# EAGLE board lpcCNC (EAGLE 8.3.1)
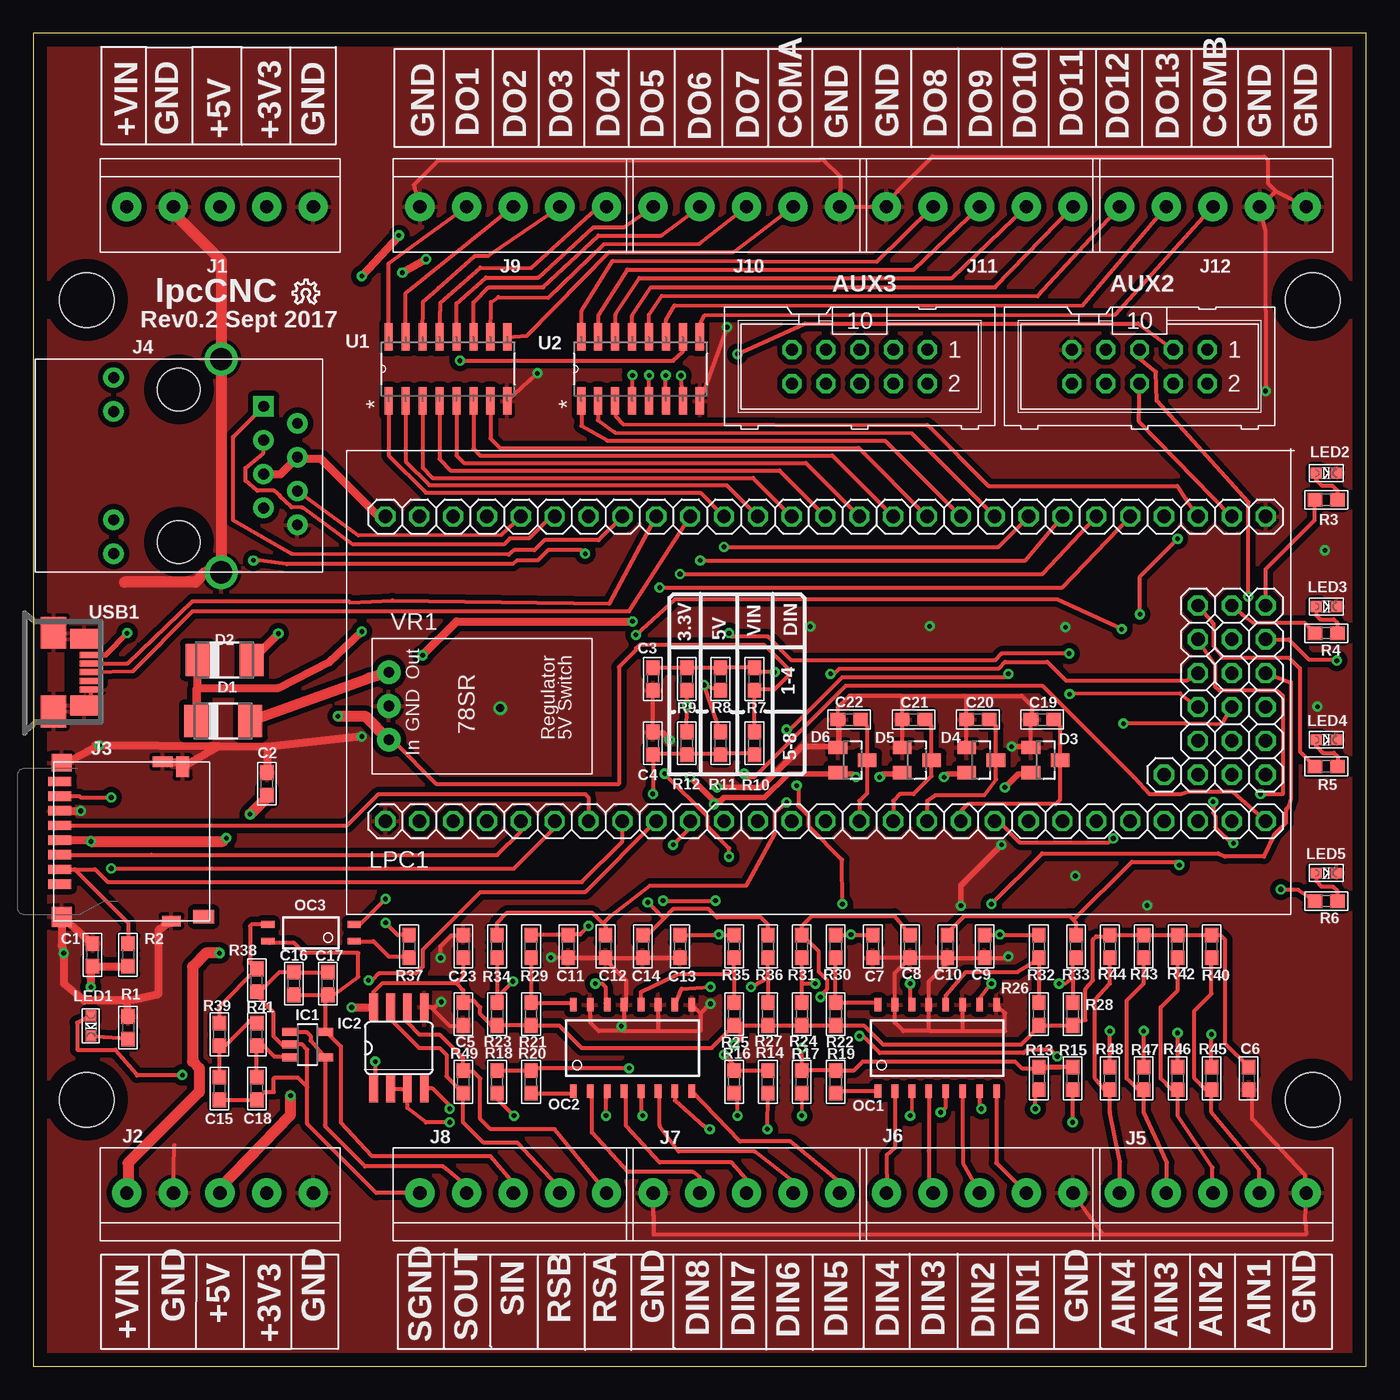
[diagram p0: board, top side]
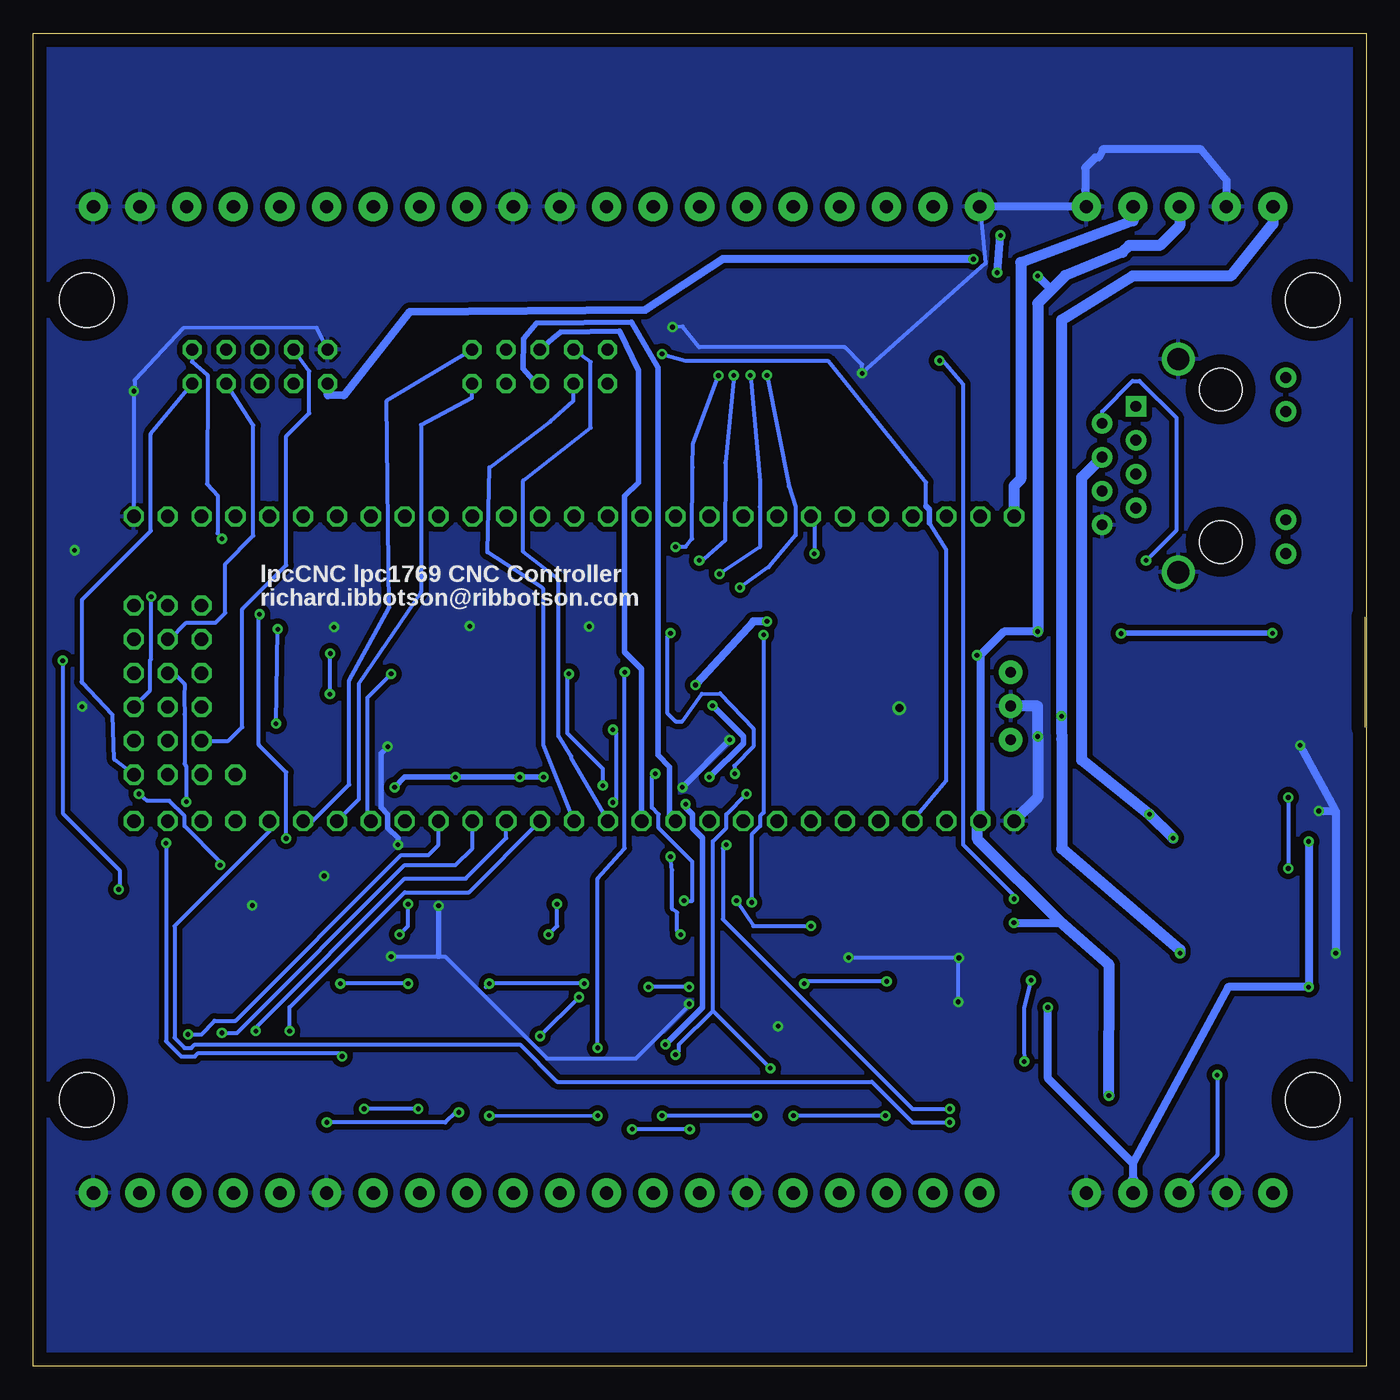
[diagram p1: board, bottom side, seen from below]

Size 100 x 100 mm. Coordinates in mm from the lower left corner, seen from the top.
Outline: 0,0 100,0 100,100 0,100 0,0
Copper layers (1*16): Top 0.035mm / dielectric 1.5mm / Bottom 0.035mm
Design rules "pcbway": minimum track width 6mil, minimum drill 0.3mm, track to track 0.205mm, track to pad 0.205mm, pad to pad 0.205mm, via to via 0.205mm, smd to smd 8mil, copper to edge 40mil, drill to drill 8mil, minimum pad ring 10mil, minimum via ring 8mil, stop-mask expansion 4mil, vias tented up to drill 25mil, thermal gap 10mil
Holes 4.1 mm at 4,20 96,20 96,80 4,80

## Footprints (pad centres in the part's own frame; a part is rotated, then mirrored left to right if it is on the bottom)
ML10 = drill 0.914 octagon: 1 -5.08,-1.27; 2 -5.08,1.27; 3 -2.54,-1.27; 4 -2.54,1.27; 5 0,-1.27; 6 0,1.27; 7 2.54,-1.27; 8 2.54,1.27; 9 5.08,-1.27; 10 5.08,1.27
0603 = smd 1.1 x 1: 1 -0.85,0; 2 0.85,0
DO-214AC = smd 1.8 x 2.4: A 2.025,0; C -2.025,0
SOT23 = smd 1 x 1.4: 1 -0.95,-1.1; 2 0.95,-1.1; 3 0,1.1
SOT23-5 = smd 0.6 x 1.2: 1 -0.95,-1.306; 2 0,-1.306; 3 0.95,-1.306; 4 0.95,1.306; 5 -0.95,1.306
SO08 = smd 0.66 x 2.032: 1 -1.905,-3.073; 2 -0.635,-3.073; 3 0.635,-3.073; 4 1.905,-3.073; 5 1.905,3.073; 6 0.635,3.073; 7 -0.635,3.073; 8 -1.905,3.073
1X05-3.5MM = drill 1 pad 2.184: 1 7,0; 2 3.5,0; 3 0,0; 4 -3.5,0; 5 -7,0
AMPHENOL_114-00841-68 = smd 0.7 x 1.75: 1 3.2,-5.888; 2 2.1,-5.888; 3 1,-5.888; 4 -0.1,-5.888; 5 -1.2,-5.888; 6 -2.3,-5.888; 7 -3.4,-5.888; 8 -4.5,-5.888 | smd 1 x 1.55: CD1 5.65,4.912 | smd 1.55 x 1: CD2 -5.602,3.337 | smd 1.3 x 1.5: SH1 -5.9,-5.76 | smd 1.5 x 1.5: SH2 5.65,-5.76 | smd 0.8 x 1.4: SH3 5.975,2.487 | smd 0.8 x 1.5: SH4 -5.975,1.837
HR911105A = drill 0.813 pad 1.524 square: 1 4.445,-6.35 | drill 0.813 pad 1.524: 2 3.175,-8.89; 3 1.905,-6.35; 4 0.635,-8.89; 5 -0.635,-6.35; 6 -1.905,-8.89; 7 -3.175,-6.35; 8 -4.445,-8.89; 9 6.604,4.902; 10 4.064,4.902; 11 -4.064,4.902; 12 -6.604,4.902 | drill 1.651 pad 2.159: 13 8.001,-3.175; 14 -8.001,-3.175 | hole 3.2: 5.715,0; -5.715,0
CHIPLED_0603 = smd 0.8 x 0.8: A 0,-0.75; C 0,0.75
LPCXPRESSO_LPC1769 = drill 1 octagon: 1 -0.635,-10.795; 2 1.905,-10.795; 3 4.445,-10.795; 4 6.985,-10.795; 5 9.525,-10.795; 6 12.065,-10.795; 7 14.605,-10.795; 8 17.145,-10.795; 9 19.685,-10.795; 10 22.225,-10.795; 11 24.765,-10.795; 12 27.305,-10.795; 13 29.845,-10.795; 14 32.385,-10.795; 15 34.925,-10.795; 16 37.465,-10.795; 17 40.005,-10.795; 18 42.545,-10.795; 19 45.085,-10.795; 20 47.625,-10.795; 21 50.165,-10.795; 22 52.705,-10.795; 23 55.245,-10.795; 24 57.785,-10.795; 25 60.325,-10.795; 26 62.865,-10.795; 27 65.405,-10.795; 28 -0.635,12.065; 29 1.905,12.065; 30 4.445,12.065; 31 6.985,12.065; 32 9.525,12.065; 33 12.065,12.065; 34 14.605,12.065; 35 17.145,12.065; 36 19.685,12.065; 37 22.225,12.065; 38 24.765,12.065; 39 27.305,12.065; 40 29.845,12.065; 41 32.385,12.065; 42 34.925,12.065; 43 37.465,12.065; 44 40.005,12.065; 45 42.545,12.065; 46 45.085,12.065; 47 47.625,12.065; 48 50.165,12.065; 49 52.705,12.065; 50 55.245,12.065; 51 57.785,12.065; 52 60.325,12.065; 53 62.865,12.065; 54 65.405,12.065; 55 57.785,-7.315; 56 60.325,-7.315; 57 62.865,-7.315; 58 65.405,-7.315; 59 60.325,-4.775; 60 62.865,-4.775; 61 65.405,-4.775; 62 60.325,-2.235; 63 62.865,-2.235; 64 65.405,-2.235; 65 60.325,0.305; 66 62.865,0.305; 67 65.405,0.305; 68 60.325,2.845; 69 62.865,2.845; 70 65.405,2.845; 71 60.325,5.385; 72 62.865,5.385; 73 65.405,5.385
MINI-FLAT-16 = smd 1 x 0.5: 1 -3.24,4.445; 2 -3.24,3.175; 3 -3.24,1.905; 4 -3.24,0.635; 5 -3.24,-0.635; 6 -3.24,-1.905; 7 -3.24,-3.175; 8 -3.24,-4.445; 9 3.24,-4.445; 10 3.24,-3.175; 11 3.24,-1.905; 12 3.24,-0.635; 13 3.24,0.635; 14 3.24,1.905; 15 3.24,3.175; 16 3.24,4.445
MINI-FLAT-4 = smd 1 x 0.5: 1 -3.24,0.635; 2 -3.24,-0.635; 3 3.24,-0.635; 4 3.24,0.635
SOIC127P600X175-16N = smd 2.057 x 0.61: 1 -4.801,8.89; 2 -4.801,7.62; 3 -4.801,6.35; 4 -4.801,5.08; 5 -4.801,3.81; 6 -4.801,2.54; 7 -4.801,1.27; 8 -4.801,0; 9 0,0; 10 0,1.27; 11 0,2.54; 12 0,3.81; 13 0,5.08; 14 0,6.35; 15 0,7.62; 16 0,8.89
MOLEX-47364-0001 = smd 1.7 x 0.45: 1 2.8,1.3; 2 2.8,0.65; 3 2.8,0; 4 2.8,-0.65; 5 2.8,-1.3 | smd 1.9 x 2.375: GND1 0,2.95; GND4 0,-2.95 | smd 2.1 x 1.475: GND2 2.3,2.5; GND3 2.3,-2.5
78SR = drill 0.8 pad 1.778: P1 -2.54,0; P2 0,0; P3 2.54,0

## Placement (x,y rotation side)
AUX2  [ML10]  83,75 180 top
AUX3  [ML10]  62,75 180 top
C1  100n  [0603]  4.45,30.86 90 top
C2  100n  [0603]  17.53,43.69 90 top
C3  100n  [0603]  46.48,51.56 270 top
C4  100n  [0603]  46.48,46.74 90 top
C5  100n  [0603]  32.26,26.42 270 top
C6  100n  [0603]  91.19,21.59 270 top
C7  100n  [0603]  62.99,31.5 270 top
C8  100n  [0603]  65.79,31.5 270 top
C9  100n  [0603]  71.37,31.5 270 top
C10  100n  [0603]  68.58,31.5 270 top
C11  100n  [0603]  40.13,31.5 270 top
C12  100n  [0603]  42.93,31.5 270 top
C13  100n  [0603]  48.51,31.5 270 top
C14  100n  [0603]  45.72,31.5 270 top
C15  47n  [0603]  13.97,20.83 270 top
C16  1uF  [0603]  19.56,28.7 90 top
C17  100n  [0603]  22.1,28.7 90 top
C18  100n  [0603]  16.76,20.83 270 top
C19  1uF  [0603]  75.69,48.51 180 top
C20  1uF  [0603]  70.87,48.51 180 top
C21  1uF  [0603]  66.04,48.51 180 top
C22  1uF  [0603]  61.21,48.51 180 top
C23  100n  [0603]  32.26,31.5 90 top
D1  [DO-214AC]  14.35,52.98 0 top
D2  [DO-214AC]  14.25,48.41 0 top
D3  BAS70  [SOT23]  75.95,45.47 270 top
D4  BAS70  [SOT23]  71.12,45.47 270 top
D5  BAS70  [SOT23]  66.29,45.47 270 top
D6  BAS70  [SOT23]  61.47,45.47 270 top
IC1  TLV172  [SOT23-5]  20.57,24.13 270 top
IC2  MAX3485  [SO08]  27.43,23.88 0 top
J1  1X5  [1X05-3.5MM]  14,87 180 top
J2  1X5  [1X05-3.5MM]  14,13 0 top
J3  [AMPHENOL_114-00841-68]  7.87,39.37 270 top
J4  HR911105A  [HR911105A]  10.92,67.56 90 top
J5  1X5  [1X05-3.5MM]  88.5,13 0 top
J6  1X5  [1X05-3.5MM]  71,13 0 top
J7  1X5  [1X05-3.5MM]  53.5,13 0 top
J8  1X5  [1X05-3.5MM]  36,13 0 top
J9  1X5  [1X05-3.5MM]  36,87 180 top
J10  1X5  [1X05-3.5MM]  53.5,87 180 top
J11  1X5  [1X05-3.5MM]  71,87 180 top
J12  1X5  [1X05-3.5MM]  88.5,87 180 top
LED1  [CHIPLED_0603]  4.32,25.53 180 top
LED2  [CHIPLED_0603]  97,67 270 top
LED3  [CHIPLED_0603]  97,57 270 top
LED4  [CHIPLED_0603]  97,47 270 top
LED5  [CHIPLED_0603]  97,37 270 top
LPC1  [LPCXPRESSO_LPC1769]  27.05,51.69 0 top
OC1  TLP293-4  [MINI-FLAT-16]  67.82,23.88 90 top
OC2  TLP293-4  [MINI-FLAT-16]  44.96,23.88 90 top
OC3  OCPL217-500E  [MINI-FLAT-4]  20.83,32.51 180 top
R1  1K  [0603]  7.11,25.4 270 top
R2  100K  [0603]  7.11,30.86 270 top
R3  1K  [0603]  97,65 0 top
R4  1K  [0603]  97,55 0 top
R5  1K  [0603]  97,45 0 top
R6  1K  [0603]  97,34.9 0 top
R7  DNF  [0603]  54.1,51.56 270 top
R8  0R  [0603]  51.56,51.56 270 top
R9  DNF  [0603]  49.02,51.56 270 top
R10  DNF  [0603]  54.1,46.74 90 top
R11  0R  [0603]  51.56,46.74 90 top
R12  DNF  [0603]  49.02,46.74 90 top
R13  470R  [0603]  75.44,21.59 90 top
R14  470R  [0603]  55.12,21.34 90 top
R15  470R  [0603]  77.98,21.59 90 top
R16  470R  [0603]  52.58,21.34 90 top
R17  470R  [0603]  57.66,21.34 90 top
R18  470R  [0603]  34.8,21.34 90 top
R19  470R  [0603]  60.2,21.34 90 top
R20  470R  [0603]  37.34,21.34 90 top
R21  2K2  [0603]  37.34,26.42 270 top
R22  2K2  [0603]  60.2,26.42 270 top
R23  2K2  [0603]  34.8,26.42 270 top
R24  2K2  [0603]  57.66,26.42 270 top
R25  2K2  [0603]  52.58,26.42 270 top
R26  2K2  [0603]  75.44,26.42 270 top
R27  2K2  [0603]  55.12,26.42 270 top
R28  2K2  [0603]  77.98,26.42 270 top
R29  1K  [0603]  37.34,31.5 90 top
R30  1K  [0603]  60.2,31.5 270 top
R31  1K  [0603]  57.66,31.5 270 top
R32  1K  [0603]  75.44,31.5 270 top
R33  1K  [0603]  78.23,31.5 270 top
R34  1K  [0603]  34.8,31.5 90 top
R35  1K  [0603]  52.58,31.5 90 top
R36  1K  [0603]  55.12,31.5 90 top
R37  470R  [0603]  28.19,31.5 270 top
R38  2K2  [0603]  16.76,28.96 90 top
R39  47K  [0603]  13.97,24.89 90 top
R40  4K7  [0603]  88.39,31.5 90 top
R41  100K  [0603]  16.76,24.89 90 top
R42  4K7  [0603]  85.85,31.5 90 top
R43  4K7  [0603]  83.31,31.5 90 top
R44  4K7  [0603]  80.77,31.5 90 top
R45  10K  [0603]  88.39,21.59 270 top
R46  10K  [0603]  85.85,21.59 270 top
R47  10K  [0603]  83.31,21.59 270 top
R48  10K  [0603]  80.77,21.59 270 top
R49  120R  [0603]  32.26,21.34 270 top
U1  ULQ2003  [SOIC127P600X175-16N]  35.56,77.22 90 top
U2  ULQ2003  [SOIC127P600X175-16N]  50,77.22 90 top
U$1  [OSHW_8X70_NOTEXT]  19.46,79.73 0 top
USB1  MOLEX-47346-0001  [MOLEX-47364-0001]  1.52,52.07 0 top
VR1  78SR  [78SR]  26.67,49.53 270 top

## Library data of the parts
AUX2 AUX3 = con-ml; OC_FARNELL: unknown; OC_NEWARK: unknown
C1-C23 LED1-LED5 R1-R49 = microbuilder
D1-D6 = diode
IC1 J3 J4 LPC1 VR1 = CNClib
IC2 = maxim; MF: MAXIM; MPN: MAX481CSA; OC_FARNELL: unknown; OC_NEWARK: 90C3817
J1 J2 J5-J12 = adafruit
OC1-OC3 = optocoupler; OC_FARNELL: unknown; OC_NEWARK: unknown
U1 U2 = Texas Instruments_By_element14_Batch_1; MPN: ULN2003ADE4; OC_FARNELL: 1125398; OC_NEWARK: 93K1078; PACKAGE: SOIC-16; SUPPLIER: Texas Instruments
U$1 = ohw-logo
USB1 = usb_con-update

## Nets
+3V3: C1.1 C2.1 C5.1 C6.1 C23.1 D3.2 D4.2 D5.2 D6.2 IC2.8 J1.4 J2.2 J3.4 J4.4 J4.5 LPC1.28 R2.2 R9.2 R12.2 R21.2 R22.2 R23.2 R24.2 R25.2 R26.2 R27.2 R28.2 R40.2 R42.2 R43.2 R44.2
+5V: AUX2.10 D1.C D2.C J1.3 J2.3 LED1.A LPC1.2 R8.2 R11.2 R37.1
+12V: J1.1 J2.5 R7.2 R10.2 VR1.P3
ANI1: J5.2 R40.1 R45.2
ANI2: J5.3 R42.1 R46.2
ANI3: J5.4 R43.1 R47.2
ANI4: J5.5 R44.1 R48.2
DI1: J6.2 OC1.8
DI2: J6.3 OC1.6
DI3: J6.4 OC1.4
DI4: J6.5 OC1.2
DI5: J7.1 OC2.8
DI6: J7.2 OC2.6
DI7: J7.3 OC2.4
DI8: J7.4 OC2.2
DO1: J9.2 U1.16
DO2: J9.3 U1.15
DO3: J9.4 U1.14
DO4: J9.5 U1.13
DO5: J10.1 U1.12
DO6: J10.2 U1.11
DO7: J10.3 U1.10
DO8: J11.2 U2.16
DO9: J11.3 U2.15
DO10: J11.4 U2.14
DO11: J11.5 U2.13
DO12: J12.1 U2.12
DO13: J12.2 U2.11
ERDN: J4.6 LPC1.32
ERDP: J4.3 LPC1.33
ETDN: J4.2 LPC1.34
ETDP: J4.1 LPC1.35
GND: AUX2.9 C1.2 C2.2 C3.2 C4.2 C5.2 C6.2 C7.2 C8.2 C9.2 C10.2 C11.2 C12.2 C13.2 C14.2 C19.2 C20.2 C21.2 C22.2 C23.2 D3.1 D4.1 D5.1 D6.1 IC2.5 J1.2 J1.5 J2.1 J2.4 J3.6 J3.CD2 J3.SH1 J3.SH2 J3.SH3 J3.SH4 J4.8 J4.13 J4.14 J5.1 J6.1 J7.5 J9.1 J10.5 J11.1 J12.4 J12.5 LED2.C LED3.C LED4.C LED5.C LPC1.1 LPC1.54 OC1.9 OC1.11 OC1.13 OC1.15 OC2.9 OC2.11 OC2.13 OC2.15 R1.1 U1.8 U2.8 USB1.5 USB1.GND1 USB1.GND2 USB1.GND3 USB1.GND4 VR1.P2
N$1: D2.A VR1.P1
N$2: LED2.A R3.2
N$3: LED3.A R4.2
N$4: LED4.A R5.2
N$5: LED5.A R6.2
N$6: LED1.C R1.2
N$9: J10.4 U1.9
N$13: J12.3 U2.9
N$15: C3.1 R7.1 R8.1 R9.1 R13.2 R15.2 R17.2 R19.2
N$16: OC2.1 R20.1
N$31: OC2.3 R18.1
N$32: OC2.5 R16.1
N$33: OC2.7 R14.1
N$38: C4.1 R10.1 R11.1 R12.1 R14.2 R16.2 R18.2 R20.2
N$42: OC1.1 R19.1
N$43: OC1.3 R17.1
N$44: OC1.5 R15.1
N$49: OC1.7 R13.1
N$66: OC1.16 R22.1 R30.2
N$67: OC1.14 R24.1 R31.2
N$71: OC2.16 R21.1 R29.1
N$72: OC2.14 R23.1 R34.1
N$73: OC2.12 R25.1 R35.1
N$74: OC2.10 R27.1 R36.1
N$75: OC1.12 R26.1 R32.2
N$85: OC3.1 R37.2
N$86: OC3.3 R38.2 R39.2
N$87: C15.1 R39.1 R41.2
N$88: C18.1 IC1.3 R41.1
N$89: OC1.10 R28.1 R33.2
P0.0: IC2.1 LPC1.9
P0.1: IC2.4 LPC1.10
P0.2: AUX3.2 LPC1.21
P0.3: AUX3.1 LPC1.22
P0.4: LPC1.38 U1.1
P0.5: LPC1.39 U1.2
P0.6: J3.2 LPC1.8 R2.1
P0.7: J3.5 LPC1.7
P0.8: J3.7 LPC1.6
P0.9: J3.3 LPC1.5
P0.10: LPC1.40 U1.3
P0.11: LPC1.41 U1.4
P0.15: AUX3.7 LPC1.13
P0.16: AUX3.8 LPC1.14
P0.17: AUX3.5 LPC1.12
P0.18: AUX3.6 LPC1.11
P0.21: IC2.2 IC2.3 LPC1.23
P0.23: C22.1 D6.3 LPC1.15 R48.1
P0.24: C21.1 D5.3 LPC1.16 R47.1
P0.25: C20.1 D4.3 LPC1.17 R46.1
P0.26: C19.1 D3.3 LPC1.18 R45.1
P1.18: LPC1.73 R3.1
P1.19: LPC1.72 R4.1
P1.20: LPC1.71 R5.1
P1.21: LPC1.70 R6.1
P1.22: AUX2.4 LPC1.69
P1.23: C10.1 LPC1.68 R33.1
P1.24: C9.1 LPC1.67 R32.1
P1.25: C8.1 LPC1.66 R31.1
P1.26: C7.1 LPC1.65 R30.1
P1.27: AUX2.5 LPC1.64
P1.28: C14.1 LPC1.63 R36.2
P1.29: C13.1 LPC1.62 R35.2
P1.30: AUX2.1 LPC1.19
P1.31: C12.1 LPC1.20 R34.2
P2.0: LPC1.42 U1.5
P2.1: LPC1.43 U1.6
P2.2: LPC1.44 U1.7
P2.3: LPC1.45 U2.1
P2.4: LPC1.46 U2.2
P2.5: LPC1.47 U2.7
P2.6: LPC1.48 U2.6
P2.7: LPC1.49 U2.5
P2.8: LPC1.50 U2.4
P2.11: LPC1.52 U2.3
P2.12: AUX2.6 LPC1.53
P2.13: C11.1 LPC1.27 R29.2
P4.28: AUX2.7 LPC1.59
P4.29: AUX2.2 LPC1.58
PWMA: OC3.2 U2.10
RESET: AUX2.3 LPC1.4
RS485A: IC2.6 J8.1 R49.1
RS485B: IC2.7 J8.2 R49.2
SGND: C15.2 C16.2 C17.2 C18.2 IC1.2 J8.5 R38.1
SIN: C16.1 C17.1 IC1.5 J8.3 OC3.4
SOUT: IC1.1 IC1.4 J8.4
UDM: LPC1.36 USB1.2
UDP: LPC1.37 USB1.3
VUSB: D1.A USB1.1

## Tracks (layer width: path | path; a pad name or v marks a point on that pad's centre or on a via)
+3V3  (via drill 0.35)
  Top 0.305: 75.57,25.57 R26.2 | 75.57,25.57 R28.2 77.98,25.79 78.94,25.98 78.94,28.29 79.5,28.96 79.5,32 79.76,32.26 80.68,32.26 R44.2 R43.2 R42.2 R40.2 89.07,32.35 89.41,32 89.41,24.22 C6.1 | 75.57,25.57 74.13,24.13 63.75,24.13 62.32,25.57 R22.2 R24.2 R27.2 53.09,25.57 R25.2 50.89,23.88 41.15,23.88 39.46,25.57 R21.2 R23.2 34.38,25.57 33.53,26.42 33.53,26.92 33.02,27.43 32.42,27.43 | 32.42,27.43 C5.1 | IC2.8 25.53,28.07 26.16,28.7 31.75,28.7 | 31.75,28.7 32.26,28.19 32.26,27.6 32.42,27.43 | C23.1 32.26,29.21 31.75,28.7 | R12.2 v49.05,49.55 R9.2 | D5.2 64.84,44.52 | 14.22,39.37 v14.48,39.62 | 17.53,42.67 C2.1
  Top 0.406: v61.72,44.2 61.47,44.45 60.45,44.45 D6.2 60.2,44.45 56.64,44.45 54.86,42.67 51.82,42.67 51.56,42.42 51.05,42.42 | D5.2 64.77,44.45 63.75,44.45 v63.5,44.2 63.75,44.2 | v68.33,44.2 68.58,44.45 69.85,44.45 D4.2 | v72.9,43.43 73.91,44.45 74.68,44.45 D3.2 | v49.28,44.2 51.05,42.42 | 53.09,25.65 53.09,25.57 53.09,24.64 v52.58,24.13 | 51.05,42.42 v51.05,42.16
  Top 0.61: v23.88,26.92 25.5,26.92 IC2.8 | R2.2 C1.1 4.41,30.01 4.32,29.03 v4.32,28.45 | J3.4 4.22,39.47 v4.32,39.37 | J4.5 18.54,66.93 19.7,68.09 | 19.7,68.09 J4.4 | LPC1.28 25.91,63.75 21.59,68.07 19.72,68.07 19.7,68.09
  Top 0.813: v16.26,41.4 17.53,42.67 | v4.32,39.37 14.22,39.37
  Bottom 0.305: 26.16,63.5 LPC1.28
  Bottom 0.406: v61.72,44.2 v63.5,44.2 v68.33,44.2 72.14,44.2 v72.9,43.43 | v49.28,44.2 46.74,46.74 46.74,47.24 v49.05,49.55 | v52.58,24.13 49.78,26.92 49.78,39.62 50.55,40.39 50.55,41.4 51.05,41.91 v51.05,42.16
  Bottom 0.61: 17.5,15.21 J2.2 | 17.5,15.21 23.88,21.59 v23.88,26.92 | v4.32,39.37 v4.32,28.45 10.36,28.45 17.5,15.21
  Bottom 0.813: J1.4 17.47,85.94 25.91,82.8 25.91,66.55 26.42,66.04 LPC1.28 | 17.5,13.94 J2.2 | v14.48,39.62 v16.26,41.4 21.34,45.47 21.34,66.67 J4.4
+5V  (via drill 0.35)
  Top 0.305: R11.2 v50.32,51.1 R8.2 | R37.1 27.34,32.35 v26.43,33.26 26.42,33.27 | LED1.A 3.29,25.77 3.3,24.13 3.3,23.75 6.16,23.75 7.71,21.94 7.78,21.82 7.81,21.84 v11.18,21.84
  Top 0.406: J2.3 14,13.39
  Top 0.61: v27.69,82.04 v29.46,83.06 | v27.43,84.84 v24.64,81.79 | v24.64,55.12 22.21,52.81 18.39,50.88 12.27,50.88 D2.C D1.C | v44.96,55.88 31.75,55.88 v29.21,53.34
  Top 0.813: 14,13.39 19.3,18.85 v19.3,20.3
  Bottom 0.305: 23.1,33.26 23,33.36 | v11.18,21.84 11.18,15.82 J2.3
  Bottom 0.406: LPC1.2 29.16,40.69
  Bottom 0.61: v26.43,33.26 23.1,33.26 | v29.46,83.06 48.26,83.06 54.1,79.25 71.75,79.1 76.68,72.82 77.9,72.85 AUX2.10 | v50.32,51.1 50.29,51.18 45.97,55.88 v44.96,55.88 | v24.64,81.79 23.62,80.77 | v27.69,82.04 v27.43,84.84 | v24.64,55.12 27.18,55.12 28.96,53.34 | 28.96,53.34 LPC1.2 | v29.21,53.34 28.96,53.34
  Bottom 0.813: v19.3,20.3 19.28,30.1 23,33.36 29.16,39.52 29.16,40.69 | J1.3 14,85.57 15.49,84.07 17.78,84.07 18.29,83.57 22.57,81.82 23.62,80.77 24.64,79.76 v24.64,55.12
+12V  (via drill 0.35)
  Top 0.305: R10.2 R7.2 54.1,50.8 55.63,50.8 56.64,51.82 56.64,52.32 54.86,54.1 45.47,54.1 45.21,53.85 45.21,53.72 43.94,52.45 43.94,43.69 30.23,43.69 27.05,46.86 VR1.P3
  Top 0.813: v13.97,30.99 12.95,30.99 11.94,29.97 11.94,22.86 12.45,22.35 12.45,20.57 7.11,15.24 7.11,13.11 J2.5 | v22.86,48.77 24.89,48.77 VR1.P3
  Bottom 0.813: J1.1 7,85.71 10.16,81.79 17.53,81.79 22.86,78.49 v22.86,48.77 22.86,47.82 22.84,47.04 22.84,38.84 13.97,31.24 v13.97,30.99
ANI1
  Top 0.305: R40.1 88.39,27.94 87.12,26.67 87.12,21.59 87.97,20.74 R45.2 88.39,19.05 91.97,14.74 J5.2
ANI2
  Top 0.305: 85.48,20.74 R46.2 | 85.48,20.74 85.43,20.74 84.58,21.59 84.58,26.92 85.85,28.19 R42.1 | J5.3 88.47,14.91 85.85,18.8 85.85,20.37 85.48,20.74
ANI3
  Top 0.305: R43.1 83.31,28.7 82.04,27.43 82.04,21.59 82.89,20.74 R47.2 83.31,19.05 85.04,15.29 J5.4
ANI4
  Top 0.305: 80.67,20.74 R48.2 | 80.67,20.74 80.35,20.74 79.65,21.59 79.65,27.48 80.77,28.7 R44.1 | J5.5 81.52,15.36 80.77,19.05 80.77,20.64 80.67,20.74
DI1
  Top 0.305: OC1.8 72.26,18.16 72.24,15.24 74.27,13.24 J6.2
DI2
  Top 0.305: OC1.6 69.72,17.65 69.75,15.24 J6.3
DI3
  Top 0.305: OC1.4 67.18,16.13 67.21,13.99 67.44,13.44 J6.4
DI4
  Top 0.305: OC1.2 64.64,16.38 64.01,15.82 64.03,13.02 J6.5
DI5
  Top 0.305: 49.47,20.64 OC2.8 53.02,16.87 56.79,16.87 60.48,13.82 J7.1
DI6
  Top 0.305: J7.2 57,13.87 54.1,16.1 48.41,16.1 46.99,18.03 46.99,20.51 OC2.6
DI7
  Top 0.305: J7.3 53.47,14.05 52.38,15.29 46.99,15.29 44.45,18.03 44.45,20.51 OC2.4
DI8
  Top 0.305: J7.4 50.02,14.17 49.48,14.58 44.6,14.58 41.91,17.53 41.91,20.51 OC2.2
DO1
  Top 0.305: U1.16 26.67,82.75 J9.2
DO2
  Top 0.305: U1.15 27.94,80.52 J9.3
DO3
  Top 0.305: U1.14 29.26,79.86 30,80.52 30.4,80.9 33.15,83.31 34.13,83.31 J9.4
DO4
  Top 0.305: U1.13 30.56,79.78 33.55,82.42 37.36,82.4 41.46,86.11 42.53,87.06 J9.5
DO5
  Top 0.305: U1.12 31.75,79.73 33.96,81.69 37.89,81.69 42.01,85.45 44.31,85.45 J10.1
DO6
  Top 0.305: U1.11 33.02,79.81 34.16,80.95 38.25,80.95 42.39,84.84 47.1,84.84 J10.2
DO7
  Top 0.305: U1.10 34.34,79.83 34.9,80.21 38.65,80.16 42.8,84.18 49.96,84.2 J10.3
DO8
  Top 0.305: U2.16 41.15,79.2 43.46,82.93 63.28,82.88 J11.2
DO9
  Top 0.305: U2.15 42.39,78.84 44.58,82.27 66.06,82.27 J11.3
DO10
  Top 0.305: U2.14 43.69,78.92 45.47,81.64 68.93,81.64 J11.4
DO11
  Top 0.305: U2.13 44.93,78.82 46.35,80.95 72.15,80.95 J11.5
DO12
  Top 0.305: U2.12 46.18,78.87 47.17,80.31 75.35,80.26 J12.1
DO13
  Top 0.305: U2.11 47.47,78.51 48.11,79.6 78.71,79.58 J12.2
ERDN
  Top 0.305: LPC1.32 35.1,62.36 24.38,62.33 J4.6
ERDP
  Top 0.305: LPC1.33 38.84,63.75 37.19,62.1 35.76,62.1 35.31,61.65 23.96,61.65 20.2,64.41 19.37,64.44 18.49,65.3 18.54,65.28 18.09,65.68 16.81,65.68 15.92,66.44 15.92,67.39 17.27,68.51 J4.3
ETDN  (via drill 0.35)
  Top 0.305: v16.51,60.45 17.02,60.45 19.02,60.17 35.97,60.2 36.32,60.45 37.85,60.45 38.61,61.21 41.15,61.21 v41.4,60.96
  Bottom 0.305: J4.2 19.81,71.63 17.53,73.91 17.02,73.91 14.22,71.12 14.22,62.74 v16.51,60.45 | v41.4,60.96 41.4,63.5 LPC1.34
ETDP
  Top 0.305: LPC1.35 42.42,61.98 38.35,61.98 37.59,61.21 36.07,61.21 35.66,60.88 19.43,60.94 14.99,63.5 14.99,69.72 J4.1
GND  (via drill 0.35, 0.6)
  Top 0.305: C11.2 C12.2 42.93,30.48 44.45,28.96 44.45,27.24 OC2.13 44.32,25.92 44.33,25.15 | C11.2 C13.2 C14.2 | OC2.15 41.78,25.78 42.42,25.15 44.33,25.15 | 50.04,26.48 50.04,25.15 46.89,25.15 | 50.04,26.48 OC2.9 | 44.33,25.15 46.89,25.15 | OC2.11 46.86,25.17 46.89,25.15 | 67.31,25.15 69.82,25.15 | 67.31,25.15 65.28,25.15 64.64,25.78 OC1.15 64.64,29.5 C8.2 | 69.82,25.15 72.9,25.15 72.9,26.48 OC1.9 | OC1.11 69.72,25.24 69.82,25.15 | 67.31,25.15 67.18,25.27 OC1.13 67.18,28.87 68.69,30.37 | C8.2 C7.2 | C8.2 68.41,30.65 68.69,30.37 | 68.69,30.37 68.83,30.23 68.83,30.39 C10.2 C9.2 73.06,30.65 v73.15,30.73 | C22.2 60.36,49.44 61.21,50.29 65.1,50.29 | D5.1 C21.2 65.19,50.2 65.1,50.29 | D4.1 C20.2 70.02,50.13 69.85,50.29 | D3.1 C19.2 74.93,48.6 74.93,49.53 74.17,50.29 69.85,50.29 | 65.1,50.29 69.85,50.29 | 80.26,9.91 95.5,9.91 95.44,10.86 J5.1 95.42,14.31 91.44,18.54 91.44,20.49 C6.2 | 80.26,9.91 79.25,11.28 79.25,11.27 J6.1 | J2.4 10.58,16.59 | J7.5 46.52,12.9 46.52,11.31 46.53,9.88 80.26,9.91 | J9.1 28.56,88.63 30.4,90.47 58.98,90.47 59.03,90.53 59.26,90.53 60.55,89.23 60.55,88.18 J10.5 J11.1 64.85,88.14 67.46,90.75 92.35,90.75 92.63,90.47 92.63,88.74 93.23,88.14 | 93.23,88.14 J12.4 92.42,85.28 v92.46,73.15 | 93.23,88.14 J12.5 | U1.8 37.21,73.94 37.26,73.99 v37.82,74.5 | v52.05,77.95 U2.8 | v50.8,27.18 50.73,27.18 50.04,26.48 | C4.2 C3.2 | USB1.5 4.32,50.2 USB1.GND3 | C11.2 38.85,30.65 38.84,30.63 v38.84,30.66 | v30.56,30.63 30.56,31.5 31.37,32.31 32.22,32.31 C23.2 | C5.2 32.22,25.53 31.24,25.53 29.82,26.95 IC2.5 30.15,26.95 30.53,27.33 v30.61,27.33
  Top 0.406: v69.6,34.54 69.6,36.07 v72.64,39.12 | v73.41,46.48 74.68,46.48 D3.1 | 69.85,46.48 D4.1 | C22.2 60.45,48.51 60.45,46.74 60.71,46.48 60.45,46.23 D6.1 60.2,46.48 57.66,46.48 54.61,43.43 v51.31,43.43 | v47.75,46.99 47.24,47.5 46.48,47.5 C4.2
  Top 0.61: v24.65,47.23 v24.64,47.24 17.53,46.46 | C1.2 4.38,31.71 J3.SH2 2.11,31.54 v2.29,30.99 2.29,28.7 3.81,27.43 7.04,27.43 | 17.53,46.46 13.91,46.51 | 13.91,46.51 J3.CD2 10.84,45.34 J3.SH4 | 2.13,45.34 J3.SH1 2.26,45.15 v4.95,46.58 | v4.95,46.58 4.67,46.58 | 13.91,46.51 v4.95,46.58 | J3.6 3.54,41.67 v3.56,41.66 | 7.04,27.43 7.75,27.56 9.4,27.94 9.4,32.69 9.56,32.85 J3.SH3 | R1.1 7.11,26.09 7.04,27.43 | 17.53,46.46 C2.2
  Top 0.813: J1.2 10.67,86.83 10.67,86.36 14.1,82.93 J4.13 J4.14 12.91,59.56 12.17,58.83 6.83,58.83
  Bottom 0.305: v52.05,77.95 51.28,78.01 50.04,76.45 39.12,76.45 37.82,75.16 v37.82,74.5 28.56,82.74 J9.1 | v73.15,30.73 69.6,30.73 69.12,30.73 61.47,23.09 54.79,23.09 50.8,27.08 v50.8,27.18 | LPC1.54 v92.46,73.15 92.41,73.2 92.41,73.97 88.77,77.88 78.74,77.9 78.13,76.73 AUX2.9 | v38.84,30.66 30.53,30.66 | 30.43,30.66 30.53,30.66 | 30.53,30.66 v30.56,30.63 30.61,30.58 v30.61,27.33
  Bottom 0.406: v69.6,34.54 69.6,30.73 | v72.64,39.12 72.64,39.62 73.41,40.39 73.41,41.4 73.91,41.91 73.91,45.97 v73.41,46.48 | v47.75,46.99 v51.31,43.43
  Bottom 0.61: J1.2 10.47,88.96 12.39,91.29 19.76,91.29 20.07,90.68 20.32,90.68 21.08,89.92 21.08,88.25 J1.5 J9.1 | v24.64,47.24 24.6,47.24 24.64,47.21 | 2.29,41.69 v2.29,30.99 | 2.29,41.69 v4.95,46.58 | v3.56,41.66 2.32,41.66 2.29,41.69
  Bottom 0.813: VR1.P2 24.64,49.53 v24.64,47.24 24.64,47.21 24.64,42.67 LPC1.1
  other vias: 35.03,49.38 78.18,36.78 83.57,34.57 67.26,55.52 77.44,55.45 58.29,55.5 44.12,25.5 96.9,61.21 96.34,49.48
  pour Top (isolate 0.406): 0,99.82 100.08,99.82 100.33,100.08 100.33,0 0,0
  pour Bottom (isolate 0.406): 0.25,0 0.25,99.06 1.02,99.82 99.06,99.82 99.57,100.33 99.57,0.51 0.76,0.51
N$1
  Top 0.813: D2.A 25.22,51.64 VR1.P1
N$2
  Top 0.305: LED2.A 96.25,66.49 96.67,66.06 97.46,66.06 97.84,65.68 R3.2
N$3
  Top 0.305: LED3.A 96.25,56.35 96.57,56.03 97.56,56.03 97.81,55.78 97.81,55.03 R4.2
N$4
  Top 0.305: LED4.A 96.25,46.52 96.75,46.02 97.59,46.02 97.87,45.74 97.87,45.02 R5.2
N$5
  Top 0.305: LED5.A 96.25,36.39 96.65,35.99 97.51,35.99 97.81,35.69 97.81,34.93 R6.2
N$6
  Top 0.305: R1.2 5.31,24.68 LED1.C
N$9
  Top 0.305: U1.9 37.03,77.32 43.21,83.59 52.52,83.59 J10.4
N$13
  Top 0.305: U2.9 50.01,78.18 50.37,78.85 81.18,78.9 J12.3
N$15  (via drill 0.35)
  Top 0.305: R13.2 R15.2 75.27,22.35 74.17,22.35 73.66,22.86 62.23,22.86 61.56,22.19 R19.2 R17.2 v57.66,23.88 | C3.1 R9.1 R8.1 R7.1 54.44,52.07 v55.63,52.07
  Bottom 0.305: v57.66,23.88 57.66,36.58 55.63,38.86 v55.63,52.07
N$16
  Top 0.305: R20.1 40.36,20.49 OC2.1
N$31  (via drill 0.35)
  Top 0.305: R18.1 34.8,20.07 v36.07,18.8 | v42.97,18.8 42.97,20.05 OC2.3
  Bottom 0.305: v36.07,18.8 v42.97,18.8
N$32  (via drill 0.35)
  Top 0.305: OC2.5 45.59,18.92 v45.72,18.8 | v52.83,18.8 52.83,20.23 R16.1
  Bottom 0.305: v45.72,18.8 v52.83,18.8
N$33  (via drill 0.35)
  Top 0.305: OC2.7 48.13,19.94 50.29,18.03 v50.75,17.78 | v55.07,17.78 R14.1
  Bottom 0.305: v50.75,17.78 v55.07,17.78
N$38  (via drill 0.35)
  Top 0.305: R18.2 R20.2 37.34,22.35 v44.7,22.35 | R14.2 R16.2 52.58,22.61 v51.82,23.37 | 49.02,45.97 51.56,45.97 | 49.02,45.97 46.48,45.97 C4.1 v46.48,42.93 | 49.02,45.97 R12.1 | 51.56,45.97 54.1,45.97 R10.1 | 51.56,45.97 R11.1
  Bottom 0.305: v46.48,42.93 48.01,41.4 48.01,40.39 49.02,39.37 49.02,26.67 | 49.02,26.67 51.56,24.13 51.56,23.62 v51.82,23.37 | 49.02,26.67 v44.7,22.35
N$42
  Top 0.305: OC1.1 60.35,20.64 R19.1
N$43  (via drill 0.35)
  Top 0.254: R17.1 v57.66,18.8 | OC1.3 65.91,18.92 v65.79,18.8
  Bottom 0.254: v65.79,18.8 v57.66,18.8
N$44  (via drill 0.35)
  Top 0.305: v68.07,19.05 68.45,19.43 OC1.5 | v77.98,18.29 R15.1
  Bottom 0.305: v68.07,19.05 68.33,19.05 69.09,18.29 77.72,18.29 77.98,18.54 v77.98,18.29
N$49  (via drill 0.35)
  Top 0.305: OC1.7 70.99,19.43 v71.12,19.3 | v75.18,19.3 75.18,20.49 R13.1
  Bottom 0.305: v71.12,19.3 74.93,19.3 75.18,19.56 v75.18,19.3
N$66
  Top 0.305: OC1.16 63.22,27.27 R22.1 R30.2
N$67  (via drill 0.35)
  Top 0.305: R24.1 57.66,28.7 | 57.66,28.7 R31.2 | 57.66,28.7 58.42,28.7 58.67,28.96 v58.67,28.7 | v65.79,28.7 65.79,27.24 OC1.14
  Bottom 0.305: v58.67,28.7 v65.79,28.7 66.04,28.45
N$71
  Top 0.305: R29.1 R21.1 40.36,27.27 OC2.16
N$72  (via drill 0.35)
  Top 0.305: R34.1 R23.1 34.8,27.69 v35.98,28.86 36.07,28.96 | v42.16,28.7 42.67,28.7 42.93,28.45 42.93,27.24 OC2.14
  Bottom 0.305: v35.98,28.86 42,28.86 v42.16,28.7
N$73
  Top 0.305: 52.58,29.75 R25.1 | 52.58,29.75 R35.1 | OC2.12 45.59,28.07 48.41,29.41 52.1,29.41 52.58,29.75
N$74  (via drill 0.35)
  Top 0.305: 55.12,29.3 R27.1 | 55.12,29.3 R36.1 | OC2.10 48.64,28.32 v50.8,28.45 | v53.85,28.45 54.77,28.96 55.12,29.3
  Bottom 0.305: v50.8,28.45 v53.85,28.45
N$75
  Top 0.305: 75.44,30.55 R26.1 | 75.44,30.55 R32.2 | OC1.12 68.45,27.81 69.95,29.57 73.85,29.57 75.44,30.55
N$85
  Top 0.305: OC3.1 25.53,31.88 26.67,30.73 28.11,30.73 R37.2
N$86
  Top 0.305: R39.2 13.97,27.01 16.73,29.77 | 16.73,29.77 R38.2 | OC3.3 16.38,33.15 16.26,33.02 16.26,30.24 16.73,29.77
N$87
  Top 0.305: C15.1 R39.1 14.39,24.04 16.26,25.91 16.6,25.91 R41.2
N$88
  Top 0.305: C18.1 R41.1 | R41.1 16.93,24.04 | R41.1 17.28,24.04 18.09,23.24 19.21,23.24 IC1.3
N$89  (via drill 0.35)
  Top 0.305: 77.98,29.16 R28.1 | 77.98,29.16 77.98,30.39 R33.2 | OC1.10 70.99,27.56 v71.88,28.7 | v76.96,28.7 77.42,28.7 77.98,29.16
  Bottom 0.305: v71.88,28.7 v76.96,28.7
P0.0  (via drill 0.35)
  Top 0.305: v25.65,22.86 25.65,20.83 IC2.1 | v25.15,28.96 25.4,28.96 25.91,29.46 28.7,29.46 29.21,29.97 29.21,31.24 33.53,35.56 41.4,35.56 LPC1.9
  Bottom 0.305: v25.65,22.86 25.68,23.9 25.68,26.87 v25.15,28.96
P0.1  (via drill 0.35)
  Top 0.305: IC2.4 29.21,20.83 29.46,21.08 29.72,20.83 29.97,20.83 31.24,19.56 v31.24,19.3 | v48.01,39.12 49.28,40.39 LPC1.10
  Bottom 0.305: v31.24,19.3 34.04,19.3 48.26,33.53 48.26,38.86 v48.01,39.12
P0.2
  Bottom 0.305: AUX3.2 67.11,72.64 70.92,70.61 70.92,58.09 75.59,51.21 75.59,42.52 LPC1.21
P0.3
  Bottom 0.305: LPC1.22 79.05,40.89 76.3,43.64 76.3,51.46 73.3,56.92 73.48,72.44 AUX3.1
P0.4
  Top 0.305: U1.1 26.67,68.33 29.46,65.53 50.04,65.53 LPC1.38
P0.5
  Top 0.305: U1.2 27.94,67.87 29.72,66.09 52.02,66.09 LPC1.39
P0.6
  Top 0.305: J3.2 3.12,37.27 | 3.12,37.27 7.11,33.27 R2.1 | 3.12,37.27 4.64,37.27 5.59,36.32 41.15,36.32 44.2,39.37 LPC1.8
P0.7
  Top 0.305: J3.5 23.55,40.57 25.91,42.93 41.4,42.93 41.66,42.67 LPC1.7
P0.8  (via drill 0.35)
  Top 0.305: J3.7 3.46,42.77 3.56,42.67 v5.84,42.67 | v5.84,37.34 36.07,37.34 39.12,40.39 LPC1.6
  Bottom 0.305: v5.84,42.67 v5.84,37.34
P0.9
  Top 0.305: J3.3 8.87,38.37 12.95,38.35 34.8,38.35 36.58,40.13 LPC1.5
P0.10
  Top 0.305: U1.3 29.21,67.41 29.97,66.65 54,66.65 LPC1.40
P0.11
  Top 0.305: U1.4 30.48,68.07 31.29,67.21 55.98,67.21 LPC1.41
P0.15
  Bottom 0.305: LPC1.13 59.64,45.62 59.64,45.74 60.6,47.27 60.6,59.03 63.25,61.09 63.25,66.45 58.19,70.41 58.19,75.34 AUX3.7
P0.16
  Bottom 0.305: LPC1.14 61.72,46.61 61.72,58.3 61.87,58.45 65.93,61.07 65.79,67.44 61.21,70.87 59.49,72.44 AUX3.8
P0.17
  Bottom 0.406: AUX3.5 61.04,77.09 60.45,77.6 56.01,77.65 54.58,74.7 54.61,72.64 54.61,66.29 55.63,65.28 55.63,53.59 54.36,52.32 LPC1.12
P0.18
  Bottom 0.406: LPC1.11 52.25,41.33 52.25,44.95 53.15,45.84 53.15,74.91 55.12,78.33 62.26,78.26 63.22,77.09 63.25,74.83 62.23,73.68 AUX3.6
P0.21  (via drill 0.35)
  Top 0.305: IC2.2 IC2.3 28.19,20.57 28.04,20.57 28.07,19.36 29.46,18.29 v31.24,18.29
  Bottom 0.305: v31.24,18.29 34.04,18.29 37.08,21.34 60.71,21.34 63.5,24.13 87.88,24.13 88.14,23.88 88.65,23.88 89.41,24.64 89.41,33.02 82.3,40.13 LPC1.23
P0.23  (via drill 0.35)
  Top 0.305: R48.1 v80.77,25.15 | LPC1.15 61.98,42.42 62.57,43.01 D6.3 62.57,48.01 C22.1
  Bottom 0.305: v80.77,25.15 80.77,26.92 72.14,35.56 67.31,35.56 LPC1.15
P0.24  (via drill 0.35)
  Top 0.305: R47.1 v83.31,25.15 | LPC1.16 64.52,42.42 65.02,42.93 66.04,42.93 67.39,44.28 D5.3 67.39,48.01 C21.1
  Bottom 0.305: v83.31,25.15 83.31,25.4 72.14,36.58 67.56,36.58 64.52,39.62 LPC1.16
P0.25  (via drill 0.35)
  Top 0.305: R46.1 v85.85,25 85.85,25.15 | LPC1.17 67.06,42.42 67.67,42.82 71.32,42.82 72.22,44.03 D4.3 72.22,48.01 C20.1
  Bottom 0.305: v85.85,25 84.72,25 72.14,37.59 68.33,37.59 67.06,38.86 LPC1.17
P0.26  (via drill 0.35)
  Top 0.305: R45.1 v88.39,24.89 | LPC1.18 69.6,41.66 70.1,42.16 76.71,42.16 77.05,42.5 D3.3 77.05,48.01 C19.1
  Bottom 0.305: v88.39,24.89 87.38,24.89 86.41,25.91 84.84,25.91 72.39,38.35 70.36,38.35 69.6,39.12 LPC1.18
P1.18
  Top 0.305: R3.1 96.14,64.99 96.14,63.48 92.46,59.79 LPC1.73
P1.19
  Top 0.305: LPC1.72 90.91,56.24 91.52,55.78 95.37,55.78 R4.1
P1.20
  Top 0.305: LPC1.71 87.35,57.06 88.54,55.7 88.54,54.06 89.2,53.16 94.21,53.16 95.02,52.35 95.02,46.13 R5.1
P1.21  (via drill 0.35)
  Top 0.305: LPC1.70 94.18,54.53 95.68,53.03 97.79,53.03 97.81,53.01 97.81,52.96 v97.79,52.93 | v93.6,35.76 94.88,35.76 R6.1
  Bottom 0.305: v97.79,52.93 97.79,41.48 93.52,37.21 93.52,35.84 v93.6,35.76
P1.22
  Bottom 0.305: LPC1.69 89.76,54.53 88.52,55.78 86.33,55.78 85.6,56.52 85.6,60.2 83.49,62.31 83.49,70.59 AUX2.4
P1.23  (via drill 0.35)
  Top 0.305: C10.1 68.58,32.51 69.85,33.78 77.72,33.78 78.04,33.47 | 78.04,33.47 78.23,33.27 R33.1 | v92.08,42.93 93.73,42.93 93.73,50.32 93.24,50.72 88.95,50.72 88.65,50.98 88.65,52.6 | v85.98,37.59 85.72,37.85 82.42,37.85 78.04,33.47 | 88.65,52.63 88.65,52.6 | 88.65,52.6 87.68,54 87.38,54.3 LPC1.68
  Bottom 0.305: v92.08,42.93 91.44,42.42 89.79,42.42 88.65,41.27 88.65,40.51 85.98,37.85 v85.98,37.59
P1.24  (via drill 0.35)
  Top 0.305: C9.1 72.52,32.35 | 72.52,32.35 R32.1 | 94.17,41.97 94.36,42.55 94.36,51.31 92.46,52.02 LPC1.67 | 94.17,41.97 93.98,41.66 | v71.88,34.67 75.69,38.48 88.9,38.48 89.41,38.23 92.33,38.23 93.09,39.88 93.98,40.77 93.98,41.66 | v72.52,32.38 72.52,32.35 | 93.98,41.66 93.98,41.78 94.17,41.97
  Bottom 0.305: v71.88,34.67 71.88,33.02 v72.52,32.38
P1.25  (via drill 0.35)
  Top 0.305: C8.1 64.6,33.78 58.42,33.78 57.66,33.02 R31.1 57.78,32.26 58.93,31.11 58.93,29.59 59.56,28.96 59.56,28.32 59.05,27.81 v59.05,27.69 | v61.98,24.77 62.23,24.77 63.5,23.5 74.3,23.5 74.55,23.75 76.33,23.75 v76.83,23.24 | v90.04,39.24 90.04,39.12 88.67,40.44 88.67,41.27 88.52,41.53 v88.52,42.34
  Bottom 0.305: v61.98,24.77 v59.05,27.69 | v76.83,23.24 77.09,23.5 87.63,23.5 87.88,23.24 88.9,23.24 90.04,24.38 v90.04,39.24 | v88.52,42.34 88.52,44.96 88.65,45.21 88.65,48.92 88.67,50.01 88.67,50.24 88.65,51.18 89.92,52.45 LPC1.66
P1.26  (via drill 0.35)
  Top 0.305: R30.1 61.34,32.35 | 61.34,32.35 C7.1 | v60.71,34.67 60.68,38 58.17,40.51 58.17,41.27 57.4,42.04 57.4,43.43 v57.28,43.56 | v61.34,32.38 61.34,32.35 | v59.82,51.94 60.07,51.94 60.45,52.32 72.39,52.32 72.9,52.83 76.07,52.83 77.47,51.44 86.54,51.44 87.38,51.87 LPC1.65
  Bottom 0.305: v60.71,34.67 60.71,33.02 v61.34,32.38 | v57.28,43.56 57.28,44.83 59.94,47.5 59.94,51.82 v59.82,51.94
P1.27  (via drill 0.35)
  Top 0.305: AUX2.5 82.98,75.59 84.23,74.6 84.28,72.44 91.16,64.82 v91.16,57.73
  Bottom 0.305: LPC1.64 92.46,49.48 91.24,50.7 91.24,52.96 91.16,53.09 v91.16,57.73
P1.28  (via drill 0.35)
  Top 0.305: 47.31,33.59 48.01,34.29 50.67,34.29 51.31,33.66 54.61,33.66 55.12,33.15 R36.2 | 47.31,33.59 46.1,32.38 45.72,32.38 C14.1 | v46.1,34.8 47.31,33.59 | v45.21,54.86 48.13,57.53 76.83,57.53 v81.66,55.3 | v81.79,48.21 86.44,48.21 88.06,48.18 88.75,48.16 89.15,48.18 LPC1.63
  Bottom 0.305: v46.1,34.8 46.1,39.88 45.47,40.51 45.47,41.27 45.21,41.53 v45.21,54.86 | v81.79,48.21 v81.66,55.3
P1.29  (via drill 0.35)
  Top 0.305: C13.1 51.44,32.35 | 51.44,32.35 R35.2 | v52.2,38.23 52.2,38.86 50.55,40.51 50.55,41.27 v47.37,44.45 | v51.44,32.38 51.44,32.35 | v52.2,54.99 52.45,54.74 55.12,54.74 56.9,52.96 72.14,52.96 72.64,53.47 v77.72,53.47 | v77.75,50.42 86.03,50.47 LPC1.62
  Bottom 0.305: v52.2,38.23 52.07,37.21 52.07,34.29 51.69,34.04 51.69,32.64 v51.44,32.38 | v47.37,44.45 47.4,45.03 45.97,46.48 45.97,47.83 48.46,50.47 49.84,50.44 51.31,48.39 51.82,48.39 52.45,49.02 52.45,54.74 v52.2,54.99 | v77.75,50.42 v77.72,53.47
P1.30  (via drill 0.35)
  Top 0.305: LPC1.19 72.39,40.89 73.99,39.29 80.7,39.29 81.03,39.62 v81.03,39.6 | v83.03,56.41 83.03,59.26 v85.85,62.08 85.95,62.18
  Bottom 0.305: v81.03,39.6 81.03,44.55 83.08,46.61 83.08,56.44 83.06,56.44 v83.03,56.41 | AUX2.1 88.09,75.36 86.92,74.35 86.97,66.19 86.16,65.3 86.18,62.48 v85.85,62.08
P1.31  (via drill 0.35)
  Top 0.305: R34.2 34.8,33.27 35.56,34.04 41.91,34.04 42.74,33.21 | 42.74,33.21 42.93,33.02 C12.1 | v73.15,51.94 72.9,51.69 60.71,51.69 56.77,47.75 v56.52,47.75 | v56.52,42.29 55.63,41.53 55.63,39.98 53.49,36.07 46.25,36.07 43.31,33.78 42.74,33.21
  Bottom 0.305: v73.15,51.94 74.93,50.16 74.93,41.15 LPC1.20 | v56.52,47.75 56.26,47.5 56.26,42.55 v56.52,42.29
P2.0
  Top 0.305: U1.5 31.75,68.33 32.31,67.77 57.96,67.77 LPC1.42
P2.1
  Top 0.305: U1.6 33.02,68.83 33.53,68.33 59.94,68.33 LPC1.43
P2.2
  Top 0.305: U1.7 34.29,69.6 35,68.89 61.92,68.89 LPC1.44
P2.3
  Top 0.305: U2.1 41.12,70.54 43.08,69.44 63.91,69.44 LPC1.45
P2.4
  Top 0.305: U2.2 42.37,70.97 43.64,70.05 65.89,70 LPC1.46
P2.5  (via drill 0.35)
  Top 0.305: v51.82,61.47 72.39,61.47 LPC1.47 | U2.7 v48.59,74.32
  Bottom 0.305: v51.82,61.47 51.05,61.47 50.56,62.09 50.54,67.44 50.52,69.16 v48.59,74.32
P2.6  (via drill 0.35)
  Top 0.305: v50.04,60.45 74.42,60.45 LPC1.48 | U2.6 v47.45,74.33
  Bottom 0.305: v47.45,74.33 48.08,67.78 48.1,61.95 49.67,60.56 v50.04,60.45
P2.7  (via drill 0.35)
  Top 0.305: v48.51,59.44 75.69,59.44 LPC1.49 | U2.5 v46.2,74.35
  Bottom 0.305: v46.2,74.35 45.47,66.41 45.48,64.49 45.48,61.45 v48.51,59.44
P2.8  (via drill 0.35)
  Top 0.305: v46.99,58.42 77.22,58.42 LPC1.50 | U2.4 v44.96,74.35
  Bottom 0.305: v44.96,74.35 43.31,66.03 42.82,64.49 42.82,62.34 44.83,59.94 v46.99,58.42
P2.11
  Top 0.305: LPC1.52 86.49,65.08 85.83,66.04 71.67,66.04 67.15,70.56 67.06,70.61 44.25,70.66 43.69,71.3 U2.3
P2.12
  Top 0.305: AUX2.6 82.96,70.87 89.89,63.75 LPC1.53
P2.13  (via drill 0.35)
  Top 0.305: v47.24,34.92 v51.18,34.92 | LPC1.27 89.97,43.1 86.67,43.1 86.08,42.93 83.74,42.93 82.55,44.2 75.69,51.05 60.96,51.05 54.1,44.2 53.59,44.2 v53.34,44.45 | R29.2 37.34,32.38 40.13,32.38 C11.1 40.26,32.38 41.02,32.38 v41.66,33.02
  Bottom 0.305: v53.34,44.45 53.59,44.2 53.59,41.91 53.09,41.4 53.09,40.39 50.55,37.85 50.55,34.92 v51.18,34.92 | v41.66,33.02 45.97,33.02 v47.24,34.92
P4.28
  Bottom 0.305: LPC1.59 85.37,46.91 84.33,47.95 84.33,56.79 81.03,60.1 81.03,69.77 79.3,71.5 79.3,74.65 AUX2.7
P4.29
  Bottom 0.305: 96.34,51.28 94.06,48.87 93.93,45.52 92.76,44.6 LPC1.58 | 96.34,51.28 96.39,51.33 | 96.34,51.28 96.34,57.51 91.19,62.66 91.19,69.95 AUX2.2
PWMA  (via drill 0.35)
  Top 0.305: OC3.2 24.51,33.15 v26.42,35.05 | v32,75.44 48.01,75.44 48.74,76.12 U2.10
  Bottom 0.305: v26.42,35.05 26.42,35.31 30.23,39.12 30.23,73.66 31.75,75.44 v32,75.44
RESET  (via drill 0.35)
  Top 0.305: v52.83,75.95 57.91,78.23 82.91,78.23 AUX2.3
  Bottom 0.305: 33.02,64.52 33.02,66.29 40.39,75.44 51.05,75.44 v52.83,75.95 | 32.77,63.25 31.5,61.21 31.5,43.94 LPC1.4
  Bottom 0.406: 33.02,64.52 32.77,64.26 32.77,63.25
RS485A
  Top 0.305: IC2.6 28.07,25.78 28.96,24.89 30.48,24.89 32.26,23.11 R49.1 32.35,22.1 33.02,22.1 33.53,21.59 33.53,18.54 34.29,17.78 39.12,17.78 42.76,13.32 J8.1
RS485B
  Top 0.305: IC2.7 26.8,26.04 28.96,23.88 30.48,23.88 30.99,23.37 30.99,21.76 R49.2 32.26,18.29 33.78,16.76 36.32,16.76 39.31,13.52 J8.2
SGND
  Top 0.305: C15.2 C18.2 17.36,20.57 18.03,20.57 18.03,21.59 18.11,21.67 19.84,21.67 20.55,20.95 | 19.7,29.55 C16.2 | 19.7,29.55 C17.2 | J8.5 25.73,13 20.55,18.19 20.55,20.95 | 19.7,29.55 19.68,29.57 18.47,29.57 17.01,28.11 R38.1 16.76,27.81 18.01,26.57 18.01,24.77 18.69,24.08 19.22,24.08 IC1.2 19.29,24.16 20.17,24.16 20.55,23.75 20.55,20.95
SIN
  Top 0.305: C16.1 C17.1 | C17.1 21.88,27.63 IC1.5 21.98,25.08 23.06,24 23.06,18.29 25.4,15.75 34.29,15.75 36.02,13.72 J8.3 | C17.1 22.52,27.85 24.38,29.21 24.38,30.99 20.32,30.99 19.56,31.75 17.71,31.75 OC3.4
SOUT
  Top 0.305: J8.4 32.46,13.56 30.73,14.99 24.89,14.99 21.89,17.98 21.88,18.07 IC1.4 20.8,24.43 20.8,24.79 20.51,25.08 IC1.1
UDM
  Top 0.305: LPC1.36 43.23,57.2 26.95,57.45 23.75,57.3 23.64,57.4 11.94,57.4 7.08,52.72 USB1.2
UDP
  Top 0.305: LPC1.37 44.7,56.64 11.95,56.64 | 11.95,56.64 11.94,56.64 | USB1.3 7.48,52.15 11.95,56.64
VUSB  (via drill 0.35)
  Top 0.406: USB1.1 5.42,53.37 v7.04,54.99 7.09,55.04
  Top 0.61: D1.A 17.2,53.77 v18.39,54.97
  Bottom 0.406: v7.04,54.99 18.36,54.99 v18.39,54.97

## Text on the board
tPlace: +VIN | GND | +5V | +3V3 | GND | GND | DO1 | DO2 | DO3 | DO4 | DO5 | DO6 | DO7 | COMA | GND | GND | DO8 | DO9 | DO10 | DO11 | DO12 | DO13 | COMB | GND | GND | lpcCNC | Rev0.2 Sept 2017 | VIN | DIN | 3.3V | 5V | 1-4 | 5-8 | SIN | GND | +5V | GND | RSB | RSA | GND | GND | GND | +VIN | +3V3 | SGND | SOUT | DIN8 | DIN7 | DIN6 | DIN5 | DIN4 | DIN3 | DIN2 | DIN1 | AIN4 | AIN3 | AIN2 | AIN1
bPlace: lpcCNC lpc1769 CNC Controller | richard.ibbotson@ribbotson.com

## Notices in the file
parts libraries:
microbuilder: This work is placed in the public domain, and may be freely used for commercial and non-commercial work with the following conditions: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
